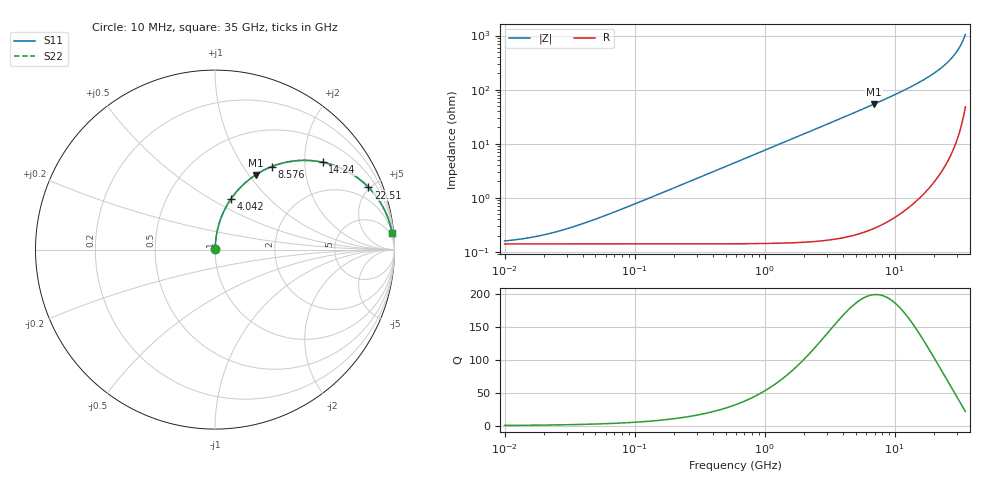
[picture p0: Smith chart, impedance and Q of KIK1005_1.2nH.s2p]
!version-3
!date-01.2023
!Series
# Hz S RI R 50
!Freq ReS11 ImS11 ReS21 ImS21 ReS12 ImS12 ReS22 ImS22
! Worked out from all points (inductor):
!   500 points, 10 MHz to 35 GHz, reference 50 ohm
!   read as one part in series: L = 1.2 nH near 56.6 MHz
!   highest Q = 199 at 6.933 GHz (marker M1), where L = 1.24 nH
!   S11 on the Smith chart (normalised r, x): 10 MHz: 1.00, +0.00; 4.042 GHz: 1.00, +0.62; 8.576 GHz: 1.01, +1.35; 14.24 GHz: 1.02, +2.45; 22.51 GHz: 1.06, +4.91; 35 GHz: 2, +21
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1e7  0.0014 0.000752  0.9986 -0.000752  0.9986 -0.000752  0.0014 0.000752
1.409773e7  0.0014 0.00106  0.9986 -0.00106  0.9986 -0.00106  0.0014 0.00106
1.955222e7  0.0014 0.00147  0.9986 -0.00147  0.9986 -0.00147  0.0014 0.00147
3.949996e7  0.00141 0.00297  0.9986 -0.00297  0.9986 -0.00297  0.00141 0.00297
6.887732e7  0.00143 0.00518  0.9986 -0.00518  0.9986 -0.00518  0.00143 0.00518
1.534938e8  0.00153 0.0115  0.9985 -0.0115  0.9985 -0.0115  0.00153 0.0115
5.964653e8  0.00342 0.0448  0.9966 -0.0448  0.9966 -0.0448  0.00342 0.0448
1.245061e9  0.0102 0.0929  0.9898 -0.0929  0.9898 -0.0929  0.0102 0.0929
2.317819e9  0.0312 0.1696  0.9688 -0.1696  0.9688 -0.1696  0.0312 0.1696
4.041653e9  0.0879 0.2802  0.9121 -0.2802  0.9121 -0.2802  0.0879 0.2802
5.33702e9  0.1449 0.3494  0.8551 -0.3494  0.8551 -0.3494  0.1449 0.3494
6.933241e9  0.226 0.4157  0.774 -0.4157  0.774 -0.4157  0.226 0.4157
8.575644e9  0.3152 0.462  0.6848 -0.462  0.6848 -0.462  0.3152 0.462
9.006867e9  0.3388 0.4707  0.6612 -0.4707  0.6612 -0.4707  0.3388 0.4707
1.151089e10  0.4716 0.4963  0.5284 -0.4963  0.5284 -0.4963  0.4716 0.4963
1.423768e10  0.5995 0.4867  0.4005 -0.4867  0.4005 -0.4867  0.5995 0.4867
1.819594e10  0.7455 0.4314  0.2545 -0.4314  0.2545 -0.4314  0.7455 0.4314
2.250634e10  0.855 0.3464  0.145 -0.3464  0.145 -0.3464  0.855 0.3464
2.565214e10  0.9093 0.2799  0.0907 -0.2799  0.0907 -0.2799  0.9093 0.2799
2.876338e10  0.9467 0.215  0.0533 -0.215  0.0533 -0.215  0.9467 0.215
3.172883e10  0.9706 0.1556  0.0294 -0.1556  0.0294 -0.1556  0.9706 0.1556
3.5e10  0.9867 0.0938  0.0133 -0.0938  0.0133 -0.0938  0.9867 0.0938
